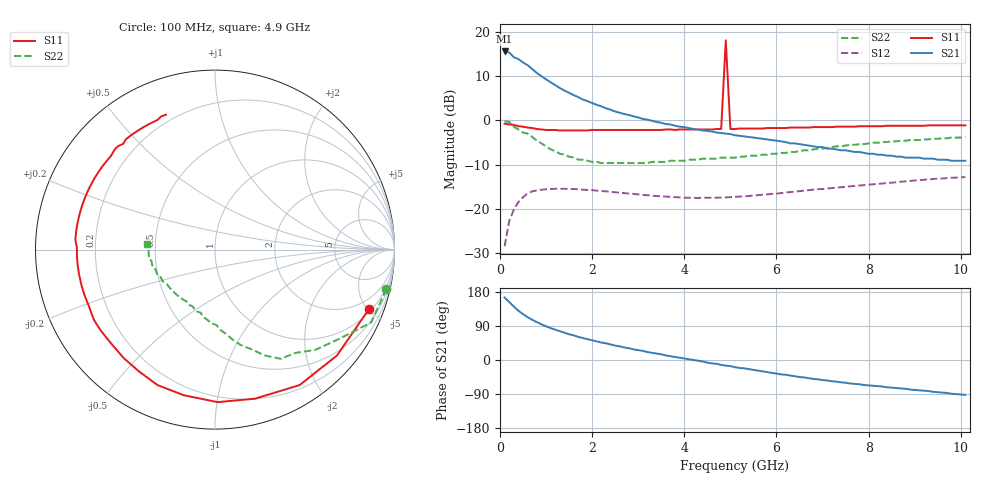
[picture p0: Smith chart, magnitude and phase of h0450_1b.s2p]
!HBFP-0450
!S and NOISE PARAMETERS at Vce=1V  Ic=2mA.  LAST UPDATED  09-04-98
# GHZ S MA R  50
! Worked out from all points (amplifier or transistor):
!   101 points, 100 MHz to 10.1 GHz, reference 50 ohm
!   highest |S21| = 15.6 dB at 100 MHz (marker M1)
!   |S21| within 3 dB of that: start of sweep to 584.6 MHz
!   unconditionally stable (mu >= 1): 3.16 GHz to 4.805 GHz; 4.994 GHz to end of sweep
!   at 1.7 GHz: K = 0.48, MSG = 10.4 dB, |S12| = -15.5 dB
!   at 5.1 GHz: K = 1.48, MAG = 2.8 dB, |S12| = -17.3 dB
!   at 10.1 GHz: K = 1.22, MAG = -1.0 dB, |S12| = -12.8 dB
!   lowest NFmin = 1.43 dB at 1.8 GHz
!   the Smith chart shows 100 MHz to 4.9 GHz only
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0.1  0.92 -21.0  6.01 165.0  0.038 78.0  0.98 -13.0
0.2  0.9 -41.0  5.86 153.0  0.073 66.0  0.96 -25.0
0.3  0.89 -58.0  5.17 141.0  0.098 55.0  0.85 -36.0
0.4  0.86 -75.0  4.93 130.0  0.12 47.0  0.79 -45.0
0.5  0.85 -89.0  4.51 121.0  0.136 39.0  0.73 -52.0
0.6  0.83 -102.0  4.21 113.0  0.15 32.0  0.71 -59.0
0.7  0.82 -113.0  3.8 106.0  0.158 27.0  0.65 -65.0
0.8  0.8 -122.0  3.43 100.0  0.162 22.0  0.59 -70.0
0.9  0.79 -130.0  3.16 94.0  0.165 18.0  0.55 -75.0
1  0.78 -138.0  2.91 89.0  0.167 14.0  0.51 -79.0
1.2  0.78 -150.0  2.5 80.0  0.169 8.0  0.45 -86.0
1.5  0.77 -165.0  2.05 68.0  0.168 1.0  0.39 -97.0
1.8  0.77 -177.0  1.72 58.0  0.165 -5.0  0.36 -106.0
2.5  0.78 161.0  1.26 38.0  0.154 -14.0  0.33 -126.0
3.5  0.78 138.0  0.94 15.0  0.139 -20.0  0.34 -152.0
4.8  0.8 110.0  0.72 -13.0  0.135 -21.0  0.38 178.0
4.9  8 107.0  0.71 -15.0  0.135 -21.0  0.38 175.0
5  0.8 105.0  0.7 -16.0  0.136 -21.0  0.38 173.0
5.1  0.8 103.0  0.68 -19.0  0.137 -22.0  0.38 171.0
6.8  0.84 68.0  0.51 -50.0  0.165 -29.0  0.47 126.0
8.5  0.87 40.0  0.4 -73.0  0.198 -45.0  0.58 90.0
10.1  0.88 15.0  0.35 -92.0  0.229 -66.0  0.65 57.0
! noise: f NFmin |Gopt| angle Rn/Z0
1.8  1.43  0.65  156  0.06
2  1.48  0.65  166  0.05
2.5  1.79  0.69  -175  0.04
3.5  2.14  0.75  -146  0.2
4  2.52  0.77  -133  0.41
5  2.98  0.79  -109  1.13
5.5  3.23  0.81  -97  1.71
7  3.84  0.85  -66  4.11
8  4.26  0.86  -49  6.01
10  4.72  0.85  -18  8.57
